PROGRAM MAIN
VAR
	S0: BOOL;
	S1: BOOL;
	L0: BOOL;
	p12_stanjeLucke_instanca: p12_stanjeLucke;
END_VAR

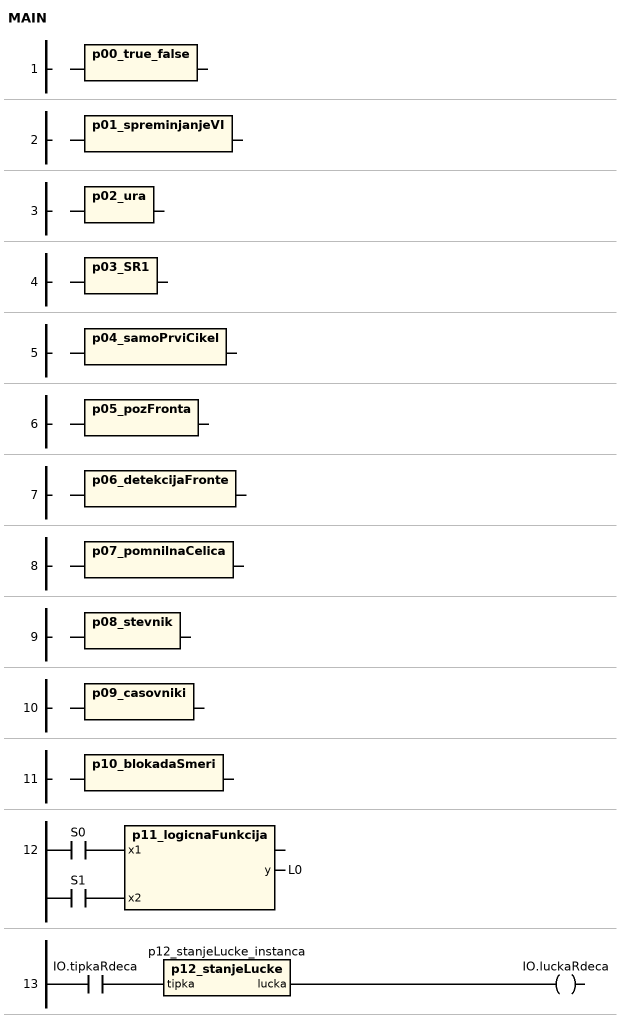
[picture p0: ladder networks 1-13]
// NETWORK 1
p00_true_false();

// NETWORK 2
p01_spreminjanjeVI();

// NETWORK 3
p02_ura();

// NETWORK 4
p03_SR1();

// NETWORK 5
p04_samoPrviCikel();

// NETWORK 6
p05_pozFronta();

// NETWORK 7
p06_detekcijaFronte();

// NETWORK 8
p07_pomnilnaCelica();

// NETWORK 9
p08_stevnik();

// NETWORK 10
p09_casovniki();

// NETWORK 11
p10_blokadaSmeri();

// NETWORK 12
p11_logicnaFunkcija(x1 := S0, x2 := S1, y => L0);

// NETWORK 13
p12_stanjeLucke_instanca(tipka := IO.tipkaRdeca); // p12_stanjeLucke
IO.luckaRdeca := p12_stanjeLucke_instanca.lucka;

END_PROGRAM
